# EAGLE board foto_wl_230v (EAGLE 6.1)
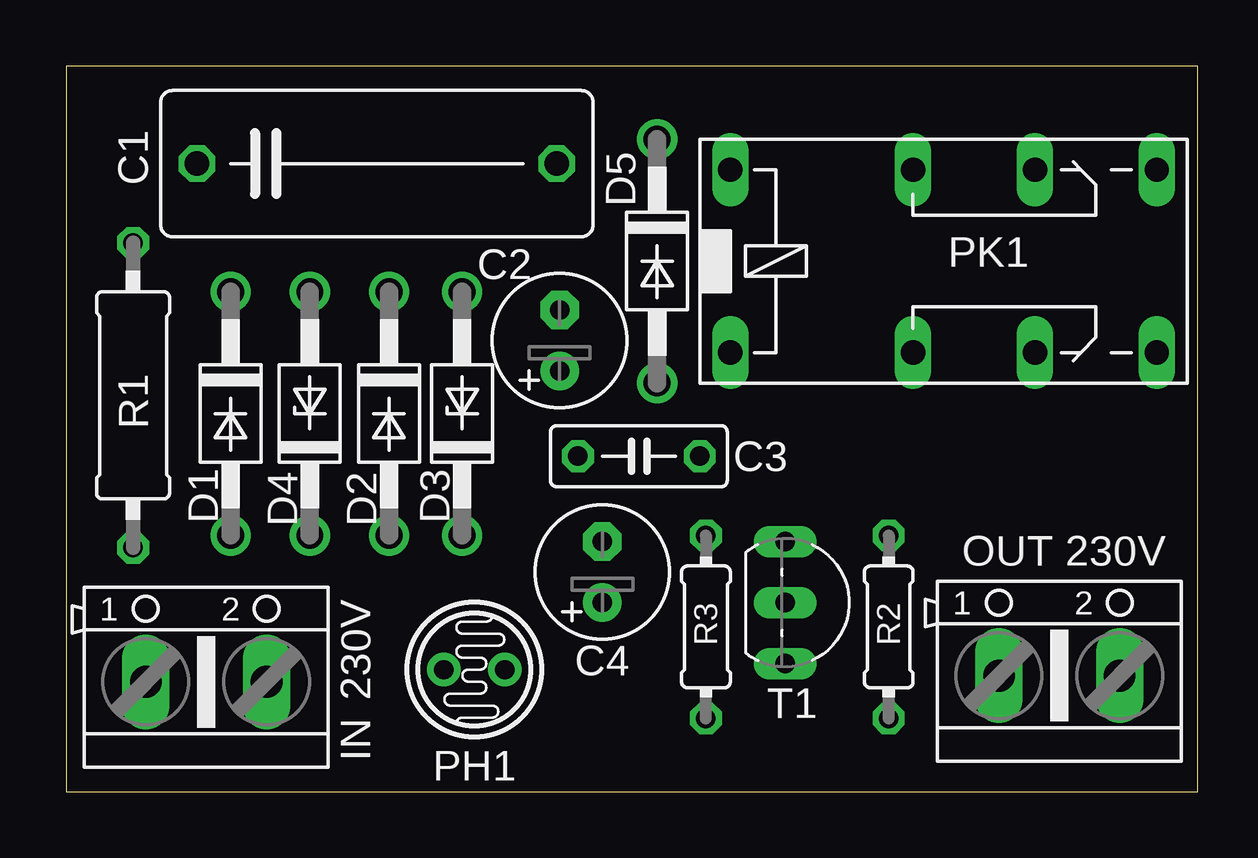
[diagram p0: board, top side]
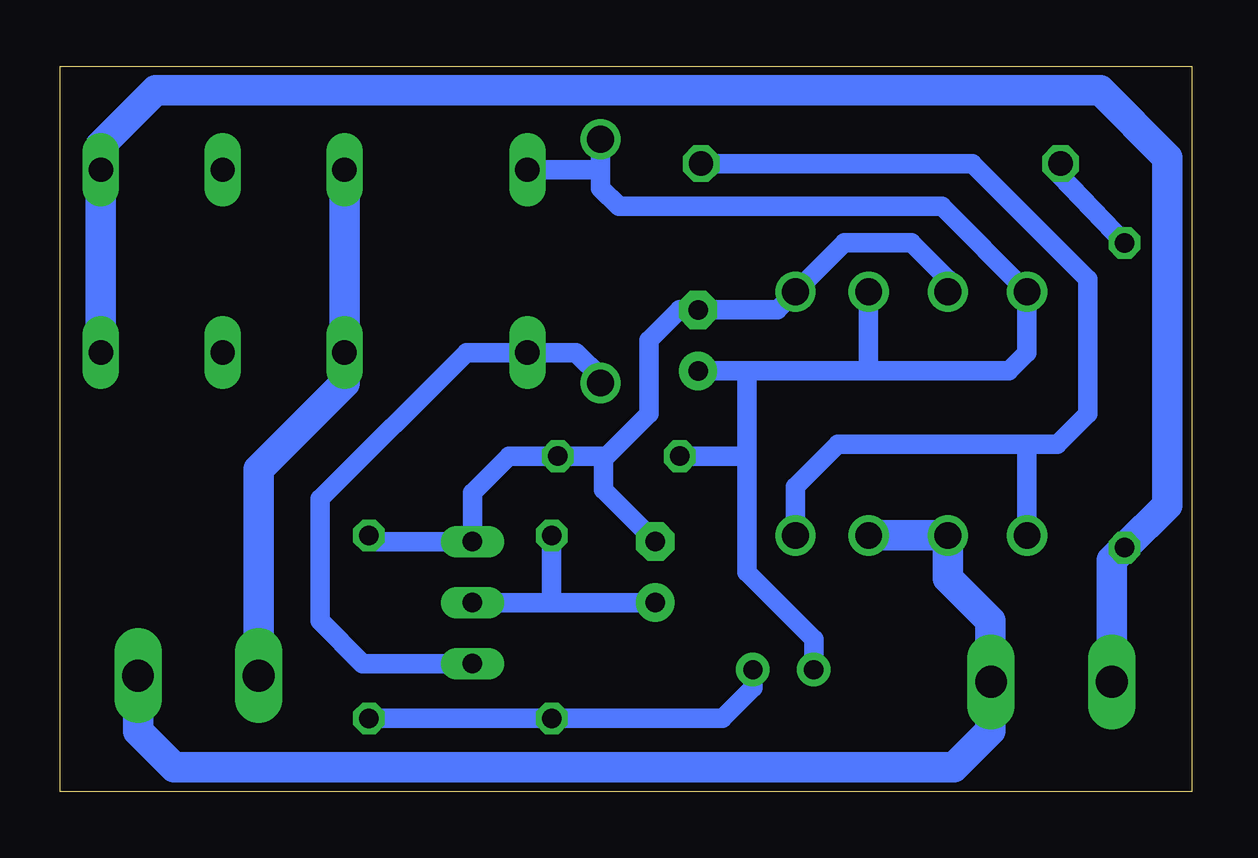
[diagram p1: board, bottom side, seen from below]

Size 47.17 x 30.22 mm. Coordinates in mm from the lower left corner, seen from the top.
Outline: 0,0 47.17,0 47.17,30.22 0,30.22 0,0
Copper layers (1*16): Top 0.035mm / dielectric 1.5mm / Bottom 0.035mm
Design rules: minimum track width 10mil, minimum drill 24mil, track to track 8mil, track to pad 8mil, pad to pad 8mil, via to via 8mil, smd to smd 8mil, copper to edge 40mil, drill to drill 8mil, minimum pad ring 10mil, minimum via ring 8mil, stop-mask expansion 4mil, vias tented up to drill 0mil, thermal gap 10mil

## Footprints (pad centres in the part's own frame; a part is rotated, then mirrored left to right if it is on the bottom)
C150-064X183 = drill 1.016 octagon: 1 -7.493,0; 2 7.493,0
E2,5-6 = drill 0.813 pad 1.6: + -1.27,0 | drill 0.813 pad 1.6 octagon: - 1.27,0
C050-025X075 = drill 0.813 octagon: 1 -2.54,0; 2 2.54,0
DO41-10 = drill 1.118: A 5.08,0; C -5.08,0
DO41Z10 = drill 1.118: A 5.08,0; C -5.08,0
AK500/2 = drill 1.321 long: 1 -2.515,0; 2 2.515,0
TO46-VT200 = drill 0.8 pad 1.4: 1 -1.27,0; 2 1.27,0
351 = drill 1.016 long: 1 -3.81,-3.81; 16 -3.81,3.81; O1 8.89,-3.81; O2 8.89,3.81; P1 3.81,-3.81; P2 3.81,3.81; S1 13.97,-3.81; S2 13.97,3.81
0309/12 = drill 0.813 octagon: 1 -6.35,0; 2 6.35,0
0204/7 = drill 0.813 octagon: 1 -3.81,0; 2 3.81,0
TO92-EBC = drill 0.813 long: B 0,-1.27; C 2.54,-1.27; E -2.54,-1.27

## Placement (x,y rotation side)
C1  470nF  [C150-064X183]  12.95,26.16 0 top
C2  220uF  [E2,5-6]  20.57,18.8 90 top
C3  100nF  [C050-025X075]  23.88,13.97 0 top
C4  100uF  [E2,5-6]  22.35,9.14 90 top
D1  1N4004  [DO41-10]  6.86,15.75 270 top
D2  1N4004  [DO41-10]  13.46,15.75 270 top
D3  [DO41Z10]  16.51,15.75 90 top
D4  [DO41Z10]  10.16,15.75 90 top
D5  1N4004  [DO41-10]  24.64,22.1 270 top
IN  [AK500/2]  5.84,4.57 0 top
OUT  [AK500/2]  41.4,4.83 0 top
PH1  [TO46-VT200]  17.02,5.08 0 top
PK1  351  [351]  31.5,22.1 0 top
R1  100/1W  [0309/12]  2.79,16.51 90 top
R2  [0204/7]  34.29,6.86 270 top
R3  [0204/7]  26.67,6.86 90 top
T1  [TO92-EBC]  31.24,7.87 270 top

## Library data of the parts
C1-C4 R1-R3 = rcl
D1-D5 = diode
IN OUT = con-ptr500; OC_FARNELL: unknown; OC_NEWARK: unknown
PH1 = photo-elements
PK1 = relay; OC_FARNELL: unknown; OC_NEWARK: unknown
T1 = transistor

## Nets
N$1: PH1.2 R2.2 R3.1
N$2: C2.+ C3.1 D1.C D2.C D5.C PH1.1 PK1.16
N$3: C2.- C3.2 C4.- D3.A D4.A R2.1 T1.E
N$4: C4.+ R3.2 T1.B
N$5: D5.A PK1.1 T1.C
N$6: OUT.1 PK1.P1
N$8: IN.1 PK1.S1 R1.1
N$9: C1.1 R1.2
N$10: C1.2 D1.A D3.C
N$11: D2.A D4.C IN.2 OUT.2

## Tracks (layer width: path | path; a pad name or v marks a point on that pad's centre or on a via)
N$1
  Bottom 0.813: PH1.2 18.29,4.32 19.56,3.05 R3.1 R2.2
N$2
  Bottom 0.813: 13.46,17.53 7.62,17.53 6.86,18.29 D1.C 10.41,24.38 23.88,24.38 24.64,25.15 24.64,25.91 | 13.46,17.53 D2.C | PH1.1 15.75,6.35 18.54,9.14 18.54,13.97 | 18.54,13.97 18.54,17.53 | D5.C 24.64,25.91 | 24.64,25.91 PK1.16 | 13.46,17.53 18.54,17.53 | 18.54,17.53 C2.+ | C3.1 18.54,13.97
N$3
  Bottom 0.813: R2.1 34.04,10.41 T1.E 29.97,12.45 28.45,13.97 C3.2 24.64,13.97 24.51,13.84 | C4.- 24.51,12.57 24.51,13.84 | 24.51,13.84 22.61,15.75 22.61,18.8 21.34,20.07 C2.- 17.27,20.07 D3.A 14.48,22.86 11.68,22.86 10.16,21.34 D4.A
N$4
  Bottom 0.813: C4.+ 26.67,7.87 | 26.67,7.87 T1.B | R3.2 26.67,7.87
N$5
  Bottom 0.813: T1.C 34.54,5.33 36.32,7.11 36.32,12.19 30.23,18.29 PK1.1 25.65,18.29 24.64,17.27 D5.A
N$6
  Bottom 1.27: OUT.1 38.89,13.44 35.31,17.02 PK1.P1 35.31,26.16
N$8
  Bottom 1.27: IN.1 3.33,9.63 R1.1 1.02,11.94 1.02,26.42 3.81,29.21 43.18,29.21 45.47,26.92 PK1.S1
N$9
  Bottom 0.813: R1.2 5.46,25.65 C1.1
N$10
  Bottom 0.813: D1.A 6.86,14.48 | 6.86,14.48 14.73,14.48 16.51,12.7 D3.C | C1.2 9.14,26.16 4.32,21.34 4.32,15.75 5.59,14.48 6.86,14.48
N$11
  Bottom 1.27: D2.A D4.C 10.16,8.89 8.38,7.11 8.38,4.6 IN.2 8.38,4.55 8.38,2.54 9.91,1.02 42.42,1.02 43.92,2.52 OUT.2

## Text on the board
tNames: OUT 230V | 230V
